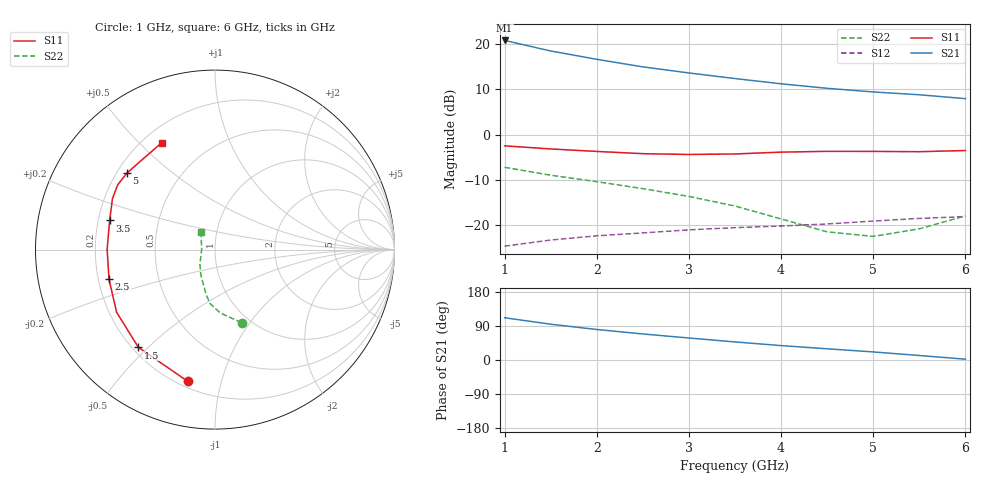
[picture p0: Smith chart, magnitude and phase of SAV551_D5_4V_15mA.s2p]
! Created Mon Oct 27 14:31:32 2008
# hz S ma R 50
! 2 Port Network Data from SP1.SP block
! freq  magS11  angS11  magS21  angS21  magS12  angS12  magS22  angS22
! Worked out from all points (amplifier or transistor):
!   11 points, 1 GHz to 6 GHz, reference 50 ohm
!   highest |S21| = 20.9 dB at 1 GHz (marker M1)
!   |S21| within 3 dB of that: start of sweep to 1.681 GHz
!   unconditionally stable (mu >= 1): 4.598 GHz to end of sweep
!   at 1.5 GHz: K = 0.46, MSG = 21.0 dB, |S12| = -23.4 dB
!   at 3.5 GHz: K = 0.89, MSG = 16.5 dB, |S12| = -20.6 dB
!   at 6 GHz: K = 1.08, MAG = 11.3 dB, |S12| = -18.2 dB
!   S11 on the Smith chart (normalised r, x): 1 GHz: 0.23, -0.79; 1.5 GHz: 0.22, -0.47; 2.5 GHz: 0.24, -0.13; 3.5 GHz: 0.25, +0.13; 5 GHz: 0.24, +0.35; 6 GHz: 0.27, +0.58
1e9  0.7494 -101.7  11.04 111.5  0.05787 39.3  0.4332 -70.0
1.5e9  0.692 -128.1  8.44 94.4  0.06767 31.2  0.3541 -85.3
2e9  0.6499 -147.5  6.819 80.5  0.07537 25.5  0.3002 -95.6
2.5e9  0.6133 -164.4  5.623 68.7  0.08111 21.1  0.2513 -101.7
3e9  0.601 179.8  4.816 58.1  0.08779 17.7  0.206 -108.1
3.5e9  0.609 164.5  4.174 47.7  0.09279 13.5  0.1613 -119.4
4e9  0.638 153.5  3.65 38.0  0.0968 10.6  0.116 -136.5
4.5e9  0.6513 146.4  3.254 29.6  0.102 8.1  0.0834 -158.4
5e9  0.6501 139.0  2.964 21.3  0.1098 5.5  0.07425 175.7
5.5e9  0.6451 128.3  2.759 11.8  0.1176 1.2  0.09009 147.9
6e9  0.6648 116.5  2.5 2.2  0.1231 -3.6  0.1253 127.7
